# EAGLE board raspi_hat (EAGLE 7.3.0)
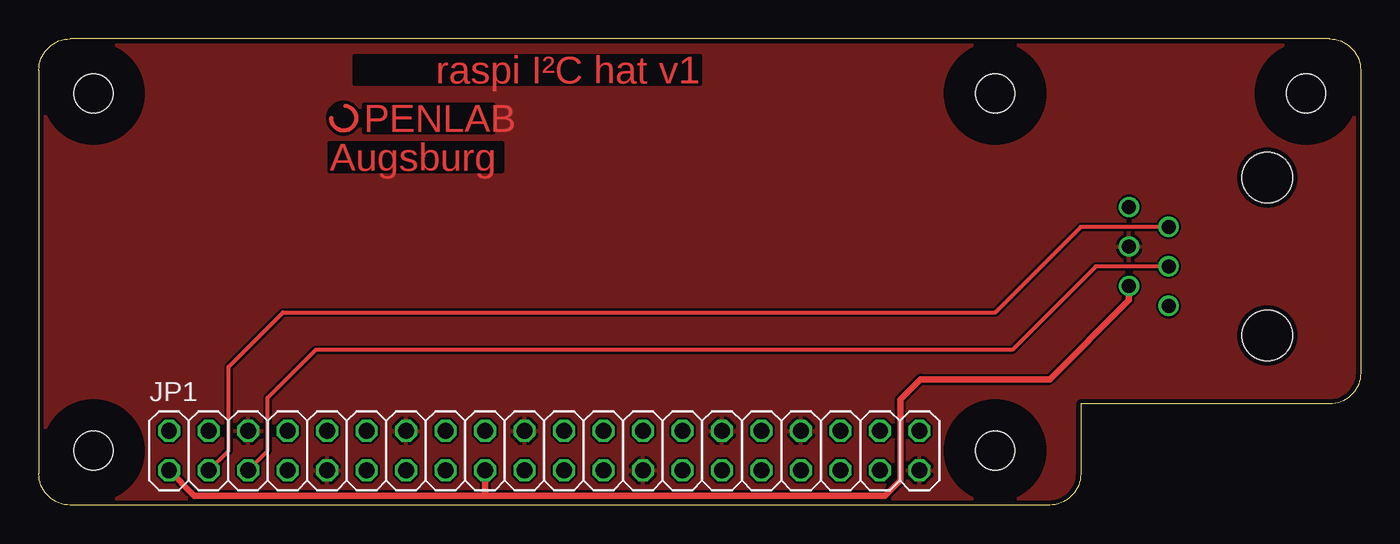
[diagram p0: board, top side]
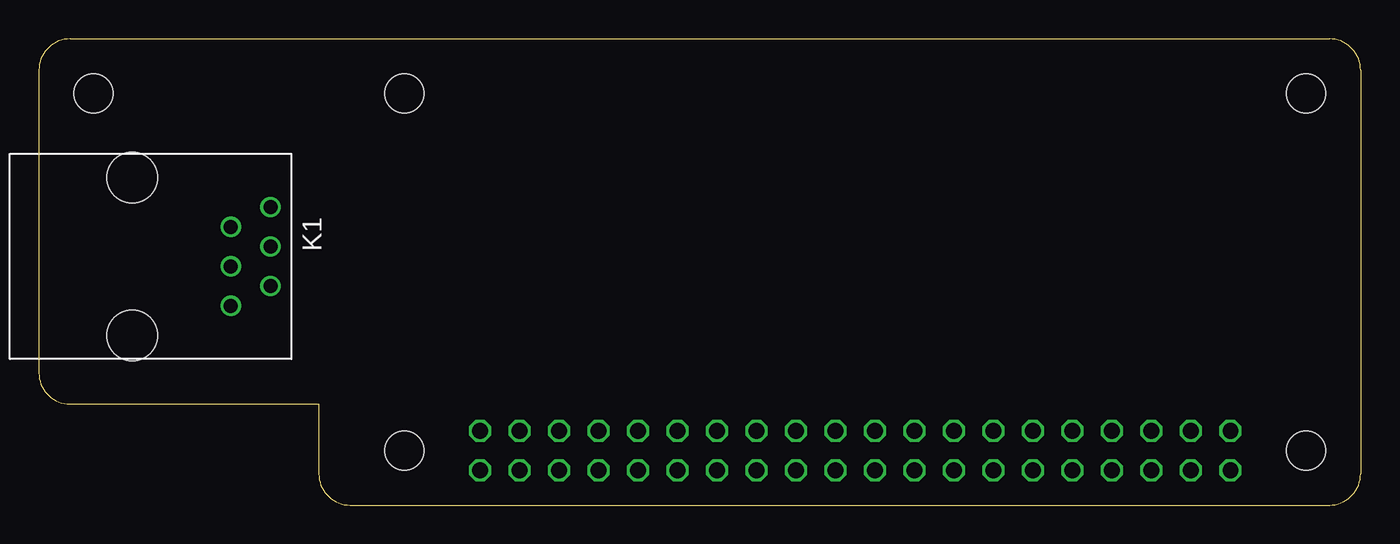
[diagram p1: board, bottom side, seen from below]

Size 85 x 30 mm. Coordinates in mm from the lower left corner, seen from the top.
Outline: 0,28 0,2 arc90 2,0 65,0 arc90 67,2 67,6.5 83,6.5 arc90 85,8.5 85,28 arc90 83,30 2,30 arc90 0,28
Copper layers (1*16): Top 0.035mm / dielectric 1.5mm / Bottom 0.035mm
Design rules "PCB-POOL Standard": minimum track width 0.15mm, minimum drill 0.3mm, track to track 0.15mm, track to pad 0.15mm, pad to pad 0.15mm, via to via 0.15mm, smd to smd 0.15mm, copper to edge 0.3mm, drill to drill 0.2mm, minimum pad ring 0.2mm, minimum via ring 0.15mm, stop-mask expansion 0.075mm, vias tented up to drill 0mil, thermal gap 0.2mm
Holes 2.5 mm at 3.5,3.5 61.5,3.5 81.5,26.5 3.5,26.5 61.5,26.5
tRestrict: area 79.2,24.2 to 83.8,28.8; area 59.2,24.2 to 63.8,28.8; area 59.2,1.2 to 63.8,5.8; area 1.2,24.2 to 5.8,28.8; area 1.2,1.2 to 5.8,5.8; area 18.6,23.9 to 20.6,25.9
bRestrict: area 79.2,24.2 to 83.8,28.8; area 59.2,24.2 to 63.8,28.8; area 59.2,1.2 to 63.8,5.8; area 1.2,24.2 to 5.8,28.8; area 1.2,1.2 to 5.8,5.8

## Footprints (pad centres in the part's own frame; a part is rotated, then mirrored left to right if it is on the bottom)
2X20 = drill 1.016 octagon: 1 -24.13,-1.27; 2 -24.13,1.27; 3 -21.59,-1.27; 4 -21.59,1.27; 5 -19.05,-1.27; 6 -19.05,1.27; 7 -16.51,-1.27; 8 -16.51,1.27; 9 -13.97,-1.27; 10 -13.97,1.27; 11 -11.43,-1.27; 12 -11.43,1.27; 13 -8.89,-1.27; 14 -8.89,1.27; 15 -6.35,-1.27; 16 -6.35,1.27; 17 -3.81,-1.27; 18 -3.81,1.27; 19 -1.27,-1.27; 20 -1.27,1.27; 21 1.27,-1.27; 22 1.27,1.27; 23 3.81,-1.27; 24 3.81,1.27; 25 6.35,-1.27; 26 6.35,1.27; 27 8.89,-1.27; 28 8.89,1.27; 29 11.43,-1.27; 30 11.43,1.27; 31 13.97,-1.27; 32 13.97,1.27; 33 16.51,-1.27; 34 16.51,1.27; 35 19.05,-1.27; 36 19.05,1.27; 37 21.59,-1.27; 38 21.59,1.27; 39 24.13,-1.27; 40 24.13,1.27
615006143621 = drill 0.9: 1 -3.175,8.89; 2 -1.905,6.35; 3 -0.635,8.89; 4 0.635,6.35; 5 1.905,8.89; 6 3.175,6.35 | hole 3.25: -5.08,0; 5.08,0

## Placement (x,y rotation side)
JP1  [2X20]  32.5,3.5 0 top
K1  615006143621  [615006143621]  79,16 270 bottom

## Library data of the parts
JP1 = pinhead
K1 = ModularJackliegendungeschirmtWR-MJ

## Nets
+3V3: JP1.1 JP1.17 K1.5
GND: JP1.6 JP1.9 JP1.14 JP1.20 JP1.25 JP1.30 JP1.34 JP1.39 K1.3
SCL: JP1.5 K1.4
SDA: JP1.3 K1.2

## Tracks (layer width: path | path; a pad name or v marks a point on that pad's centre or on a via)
+3V3
  Top 0.406: 28.6,0.6 54.4,0.6 55.4,1.6 55.4,6.8 56.7,8.1 65,8.1 70.11,13.21 K1.5 | 28.6,0.6 10,0.6 JP1.1 | JP1.17 28.69,0.69 28.6,0.6
GND
  pour Top: 85,30 85,6.5 67,6.5 67,0 0,0 0,30
N$1
  Top 0.254: 19.7,25.7 arc-263 18.8,24.9
SCL
  Top 0.254: JP1.5 13.45,2.25 14.7,3.5 14.7,6.9 17.8,10 62.6,10 67.97,15.37 K1.4
SDA
  Top 0.254: JP1.3 10.93,2.23 12.2,3.5 12.2,8.9 15.7,12.4 61.5,12.4 67,17.91 K1.2

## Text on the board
Top: raspi I²C hat v1 | PENLAB | Augsburg
tStop: raspi I²C hat v1 | PENLAB | Augsburg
